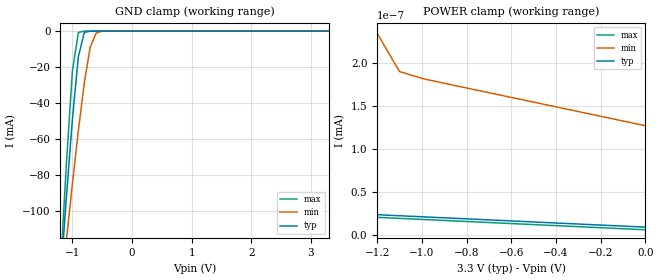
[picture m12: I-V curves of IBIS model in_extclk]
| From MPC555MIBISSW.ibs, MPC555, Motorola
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| in_extclk
[Model]   in_extclk
Model_type   Input
Polarity   Non-Inverting
|   typ   min   max
C_comp   4.7270e-13   4.1940e-13   5.4410e-13
| CAP models
| typical : model= typ
| maximum : model= wcs
| minimum : model= bcs
[Voltage range]   3.3v   3.0v   3.6v
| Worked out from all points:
|   GND clamp passes 1 mA (typ) near -0.80 V on its own axis
|   POWER clamp passes 1 mA (typ) near -2.51 V on its own axis
|  typical: model = typ,  temp = 25,  vdd = 3.3
|  maximum: model = bcs,  temp = -40, vdd = 3.6
|  minimum: model = wcs,  temp = 150, vdd = 3.0
[GND_clamp]
|  Voltage   I(typ)   I(min)   I(max)
-3.3V     -1.185A    -863.2mA   -1.512A
-1.2V     -138.1mA   -148.2mA   -133mA
-1.1V     -92.22mA   -116.2mA   -73.74mA
-1V       -49.26mA   -85.1mA    -22.51mA
-900mV    -14.32mA   -55.46mA   -776.8uA
-800mV    -817uA     -28.76mA   -5.674uA
-700mV    -17.72uA   -8.803mA   -39.16nA
-600mV    -362.1nA   -1.041mA   -309.8pA
-500mV    -7.421nA   -72.32uA   -40.86pA
-400mV    -185.5pA   -4.683uA   -37.81pA
3.3V      9.639pA    127.3pA    6.6pA
[POWER_clamp]
-3.3V     323.1mA    441.8mA    66.27mA
-2.9V     130.2mA    306.1mA    20.19nA
-2.8V     84.66mA    272.4mA    179.1pA
-2.7V     42.52mA    239mA      39.96pA
-2.2V     3.84nA     77.78mA    33pA
-2.1V     112.5pA    48.67mA    31.8pA
-2V       35.27pA    23.09mA    30.6pA
-1.3V     25.27pA    843.2pA    22.2pA
-1.2V     24.07pA    234.5pA    21pA
-1.1V     22.87pA    190.2pA    19.8pA
-1V       21.66pA    182.2pA    18.6pA
0V        9.639pA    127.3pA    6.6pA
